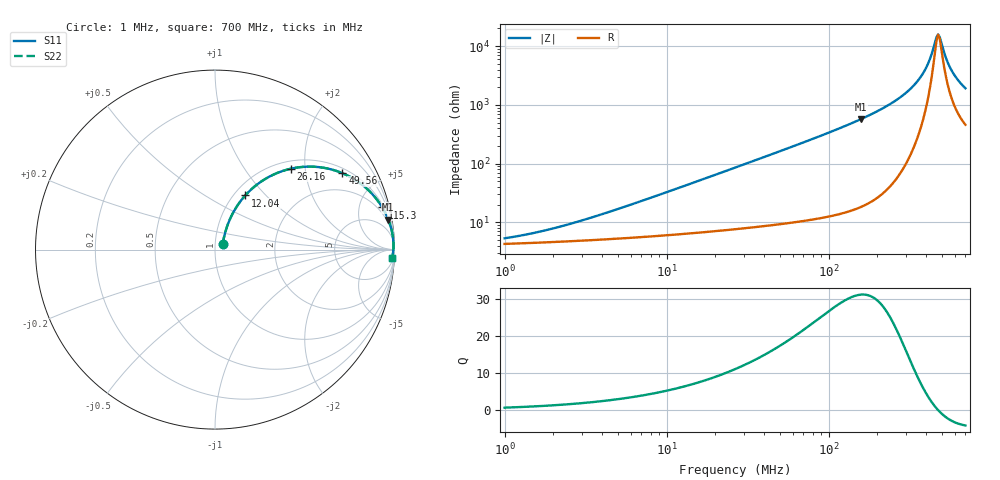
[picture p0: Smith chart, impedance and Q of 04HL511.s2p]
! Coilcraft 0402HL-511 Chip Inductor
! 20 July 2012
# MHz S MA R 50
!Freq  MagS11  AngS11  MagS21  AngS21  MagS12  AngS12  MagS22  AngS22
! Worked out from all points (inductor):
!   288 points, 1 MHz to 700 MHz, reference 50 ohm
!   read as one part in series: L = 510 nH near 4.942 MHz
!   highest Q = 31.2 at 158.8 MHz (marker M1), where L = 574 nH
!   self-resonance near 474.9 MHz
!   S11 on the Smith chart (normalised r, x): 1 MHz: 1.09, +0.06; 12.04 MHz: 1.13, +0.77; 26.16 MHz: 1.15, +1.68; 49.56 MHz: 1.19, +3.21; 115.3 MHz: 1.27, +7.85; 700 MHz: 10, -37
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1  0.05139 34.9  0.9583 -1.8  0.9583 -1.8  0.05139 34.9
2.991129  0.1021 57.8  0.9495 -5.2  0.9495 -5.2  0.1021 57.8
8.946856  0.2669 63.2  0.9115 -15.2  0.9115 -15.2  0.2669 63.2
12.03767  0.3459 60.8  0.8844 -20.0  0.8844 -20.0  0.3459 60.8
26.15727  0.6182 46.8  0.7323 -38.0  0.7323 -38.0  0.6182 46.8
26.7612  0.6267 46.3  0.7256 -38.6  0.7256 -38.6  0.6267 46.3
49.56361  0.8281 30.9  0.5149 -55.8  0.5149 -55.8  0.8281 30.9
80.04622  0.9224 20.4  0.3491 -67.2  0.3491 -67.2  0.9224 20.4
115.3327  0.9611 14.2  0.2446 -73.8  0.2446 -73.8  0.9611 14.2
158.7588  0.9798 9.8  0.1711 -78.3  0.1711 -78.3  0.9798 9.8
239.4286  0.9915 5.5  0.0965 -82.2  0.0965 -82.2  0.9915 5.5
307.7667  0.9944 3.4  0.05875 -82.8  0.05875 -82.8  0.9944 3.4
369.426  0.995 1.9  0.03374 -80.4  0.03374 -80.4  0.995 1.9
414.089  0.9947 1.0  0.01903 -73.3  0.01903 -73.3  0.9947 1.0
433.4312  0.9944 0.7  0.01352 -65.4  0.01352 -65.4  0.9944 0.7
464.1516  0.9939 0.2  0.006987 -29.7  0.006987 -29.7  0.9939 0.2
474.8682  0.9937 0.0  0.006296 -4.9  0.006296 -4.9  0.9937 0.0
485.8322  0.9935 -0.1  0.006933 20.2  0.006933 20.2  0.9935 -0.1
532.2789  0.9923 -0.8  0.01606 61.1  0.01606 61.1  0.9923 -0.8
570.0054  0.9912 -1.3  0.02453 68.4  0.02453 68.4  0.9912 -1.3
624.4992  0.9894 -2.0  0.03629 72.0  0.03629 72.0  0.9894 -2.0
700  0.9864 -2.9  0.05144 73.3  0.05144 73.3  0.9864 -2.9
